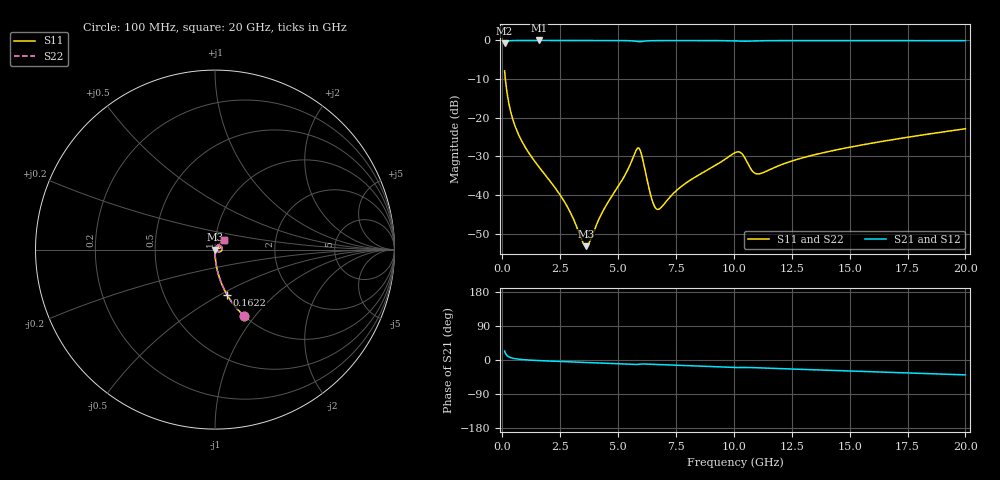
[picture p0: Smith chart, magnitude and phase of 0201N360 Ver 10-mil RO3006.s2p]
# GHz S MA R 50
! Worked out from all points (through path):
!   1601 points, 100 MHz to 20 GHz, reference 50 ohm
!   highest |S21| = -0.01 dB at 1.58 GHz (marker M1); lowest = -0.8 dB at 100 MHz (marker M2)
!   group delay of S21, straight-line fit = 5.77 ps
!   lowest |S11| = -53.2 dB at 3.62 GHz (marker M3), VSWR 1.00, Z = 50.2 - j0.0369 ohm
!   |S11| at or under -10 dB: 132.2 MHz to end of sweep
!   |S22| runs from -53.2 to -7.9 dB; largest |S21 - S12| = 0
!   S11 on the Smith chart (normalised r, x): 100 MHz: 1.00, -0.88; 162.2 MHz: 1.00, -0.54; 20 GHz: 1.10, +0.12
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0.1  0.4031 -66.3  0.9146 23.6  0.9146 23.6  0.4031 -66.3
0.1621875  0.2618 -75.0  0.9645 14.9  0.9645 14.9  0.2618 -75.0
0.34875  0.1244 -83.2  0.9915 6.5  0.9915 6.5  0.1244 -83.2
0.6099375  0.07026 -86.4  0.9967 2.9  0.9967 2.9  0.07026 -86.4
0.9955  0.04125 -88.0  0.9981 0.6  0.9981 0.6  0.04125 -88.0
1.580062  0.02313 -88.2  0.9984 -1.5  0.9984 -1.5  0.02313 -88.2
2.724312  0.007813 -81.1  0.9981 -4.5  0.9981 -4.5  0.007813 -81.1
3.420812  0.002672 -44.7  0.9978 -6.1  0.9978 -6.1  0.002672 -44.7
3.619813  0.002179 -9.7  0.9977 -6.5  0.9977 -6.5  0.002179 -9.7
4.366062  0.006352 57.0  0.9972 -8.2  0.9972 -8.2  0.006352 57.0
5.846125  0.04036 17.6  0.9644 -11.6  0.9644 -11.6  0.04036 17.6
6.02025  0.03284 -18.6  0.9673 -10.5  0.9673 -10.5  0.03284 -18.6
6.492875  0.008192 -20.0  0.9917 -11.6  0.9917 -11.6  0.008192 -20.0
6.741625  0.006526 13.9  0.994 -12.3  0.994 -12.3  0.006526 13.9
7.836125  0.01363 57.7  0.9956 -14.8  0.9956 -14.8  0.01363 57.7
10.05  0.0353 42.6  0.9828 -19.8  0.9828 -19.8  0.0353 42.6
10.33606  0.03454 25.2  0.975 -19.9  0.975 -19.9  0.03454 25.2
10.78381  0.02069 20.8  0.984 -20.0  0.984 -20.0  0.02069 20.8
11.03256  0.01874 33.7  0.9887 -20.6  0.9887 -20.6  0.01874 33.7
13.37081  0.03254 55.8  0.9943 -25.6  0.9943 -25.6  0.03254 55.8
16.69162  0.05105 52.0  0.9934 -32.4  0.9934 -32.4  0.05105 52.0
20  0.07195 46.5  0.9916 -39.3  0.9916 -39.3  0.07195 46.5
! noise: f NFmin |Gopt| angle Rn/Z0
0.1  0.0004963  0.9143  0.2815  0.001276
2.301  0.003854  0.7658  4.166  0.003342
4.515  0.007092  0.7525  8.098  0.005754
6.729  0.01251  0.7873  12.07  0.01197
8.943  0.01314  0.739  15.95  0.009889
11.14  0.02048  0.7866  19.86  0.01916
13.36  0.01602  0.6918  23.64  0.009717
15.57  0.01719  0.6712  27.4  0.009519
17.79  0.01878  0.6605  31.12  0.009848
20  0.02046  0.6535  34.78  0.01028
